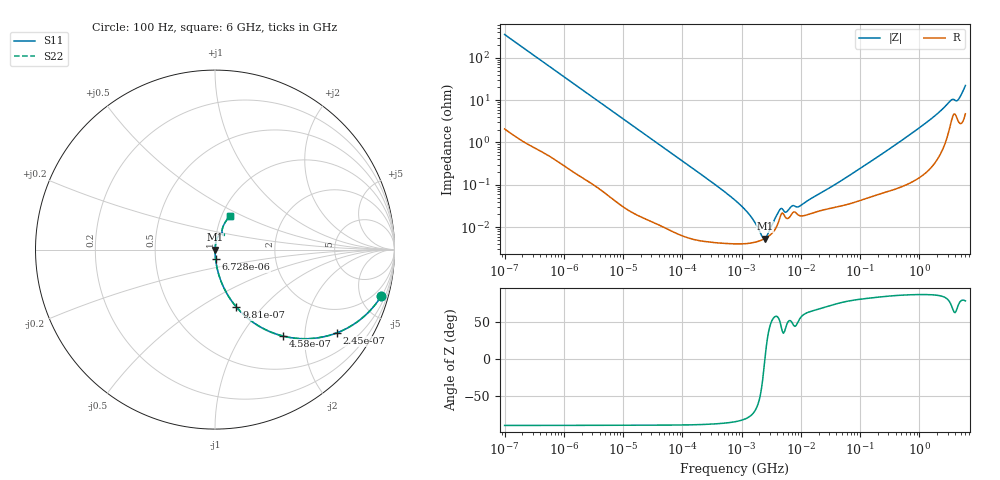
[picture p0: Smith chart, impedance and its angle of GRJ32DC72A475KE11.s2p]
!Murata Part Number: GRJ32DC72A475KE11
!These Parameters are Measured in Series Mode Connection
!Data Generated on Jun 19, 2026
!  o--ll--o
!Port1  Port2
!  o------o
!Operation Temp=25[degC], DC Bias Voltage=0[V]
!Freq. Start=100[Hz] Stop=6[GHz] 401[Steps]
# Hz S RI R 50
!Freq.(Hz) S11(Real) S11(Imag) S21(Real) S21(Imag) S12(Real) S12(Imag) S22(Real) S22(Imag)
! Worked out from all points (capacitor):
!   401 points, 100 Hz to 6 GHz, reference 50 ohm
!   read as one part in series: C = 4.47 uF near 109 Hz
!   lowest |Z| = 5.39 mohm at 2.481 MHz (marker M1)
!   series resonance near 2.48 MHz, so ESL is about 920 pH
!   S11 on the Smith chart (normalised r, x): 100 Hz: 1.04, -7.10; 245 Hz: 1.02, -2.91; 458 Hz: 1.01, -1.56; 981 Hz: 1.01, -0.73; 6.728 kHz: 1.00, -0.11; 6 GHz: 1.10, +0.43
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100  0.9252 -0.2601  0.0748 0.2601  0.0748 0.2601  0.9252 -0.2601
245  0.6781 -0.4641  0.3219 0.4641  0.3219 0.4641  0.6781 -0.4641
458  0.3787 -0.4814  0.6213 0.4814  0.6213 0.4814  0.3787 -0.4814
981  0.1198 -0.3208  0.8802 0.3208  0.8802 0.3208  0.1198 -0.3208
2008  0.0325 -0.1731  0.9675 0.1731  0.9675 0.1731  0.0325 -0.1731
6728  0.00335 -0.0537  0.9967 0.0537  0.9967 0.0537  0.00335 -0.0537
40335  0.000195 -0.00906  0.9998 0.00906  0.9998 0.00906  0.000195 -0.00906
774597  4.05e-05 -0.000433  1 0.000433  1 0.000433  4.05e-05 -0.000433
1212075  4.1e-05 -0.000235  1 0.000235  1 0.000235  4.1e-05 -0.000235
1896632  4.62e-05 -8.29e-05  1 8.29e-05  1 8.29e-05  4.62e-05 -8.29e-05
2481164  5.39e-05 1e-07  0.9999 -1e-07  0.9999 -1e-07  5.39e-05 1e-07
3103719  6.7e-05 7.22e-05  0.9999 -7.22e-05  0.9999 -7.22e-05  6.7e-05 7.22e-05
4440638  0.000168 0.0002  0.9998 -0.0002  0.9998 -0.0002  0.000168 0.0002
5809218  0.000161 0.000168  0.9998 -0.000168  0.9998 -0.000168  0.000161 0.000168
6948629  0.0002 0.000236  0.9998 -0.000236  0.9998 -0.000236  0.0002 0.000236
9506416  0.000187 0.00025  0.9998 -0.00025  0.9998 -0.00025  0.000187 0.00025
1.555665e7  0.000215 0.000443  0.9998 -0.000443  0.9998 -0.000443  0.000215 0.000443
3.124326e8  0.00076 0.00699  0.9992 -0.00699  0.9992 -0.00699  0.00076 0.00699
1.431855e9  0.00323 0.0321  0.9968 -0.0321  0.9968 -0.0321  0.00323 0.0321
3.352442e9  0.0331 0.0876  0.9669 -0.0876  0.9669 -0.0876  0.0331 0.0876
4.385646e9  0.0418 0.084  0.9582 -0.084  0.9582 -0.084  0.0418 0.084
6e9  0.0846 0.1893  0.9154 -0.1893  0.9154 -0.1893  0.0846 0.1893
